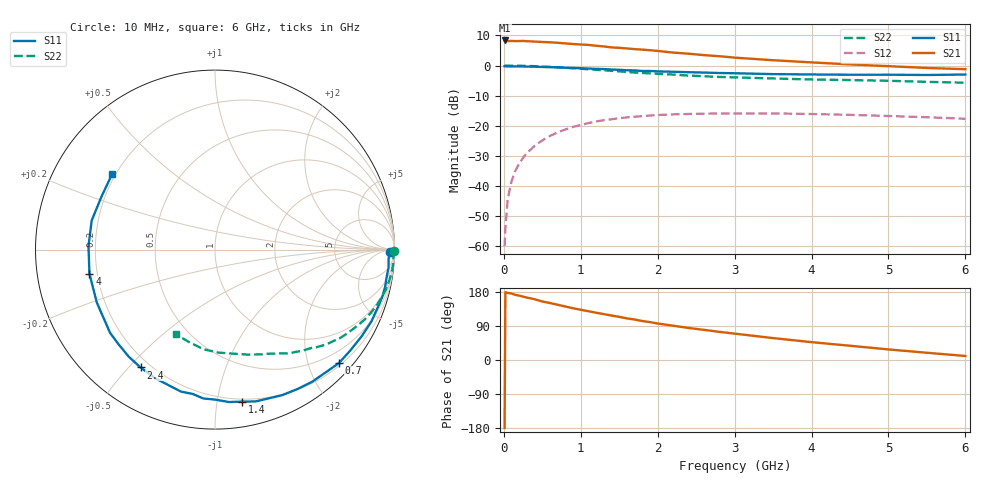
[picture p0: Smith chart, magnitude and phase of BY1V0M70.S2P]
! SIEMENS Small Signal Semiconductors
! BFY420
! Si NPN RF SIEGET Grounded Emitter Transistor in MICRO-X
! VCE = 1 V  IC = 0.7 mA
! Common Emitter S-Parameters:  October  1996
# GHz  S  MA  R  50
!  f  S11  S21  S12  S22
! GHz  MAG  ANG  MAG  ANG  MAG  ANG  MAG  ANG
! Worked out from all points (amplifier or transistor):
!   36 points, 10 MHz to 6 GHz, reference 50 ohm
!   highest |S21| = 8.4 dB at 10 MHz (marker M1)
!   |S21| within 3 dB of that: start of sweep to 1.772 GHz
!   unconditionally stable (mu >= 1): 4.688 GHz to end of sweep
!   at 250 MHz: K = 0.04, MSG = 19.4 dB, |S12| = -30.7 dB
!   at 1.4 GHz: K = 0.22, MSG = 11.9 dB, |S12| = -17.8 dB
!   at 6 GHz: K = 1.34, MAG = 4.7 dB, |S12| = -17.7 dB
!   S11 on the Smith chart (normalised r, x): 10 MHz: 60, -32; 700 MHz: 0.25, -2.55; 1.4 GHz: 0.18, -1.18; 2.4 GHz: 0.16, -0.54; 4 GHz: 0.17, -0.09; 6 GHz: 0.19, +0.32
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0.01  0.9745 -0.8  2.616 -179.4  0.001 107.4  0.9985 -0.3
0.02  0.973 -1.5  2.609 178.7  0.002 85.0  0.9984 -0.6
0.05  0.9682 -3.1  2.555 177.1  0.006 87.8  0.9968 -1.6
0.1  0.9723 -6.1  2.57 175.5  0.012 86.9  0.994 -3.3
0.15  0.9683 -9.1  2.551 171.8  0.0179 83.2  0.9947 -5.0
0.25  0.9691 -15.4  2.57 167.3  0.0293 79.3  0.9896 -8.2
0.4  0.9592 -24.6  2.506 160.4  0.0464 74.1  0.978 -13.1
0.5  0.9487 -30.9  2.469 154.4  0.0572 70.3  0.9652 -16.2
0.7  0.9361 -42.5  2.394 145.7  0.0777 63.1  0.9369 -22.1
0.9  0.9137 -53.8  2.282 136.5  0.0957 55.3  0.9025 -27.6
1.1  0.8933 -65.1  2.206 128.7  0.1109 48.6  0.8685 -32.9
1.4  0.8602 -79.9  2.005 117.3  0.1284 39.4  0.8191 -39.7
1.6  0.8357 -89.9  1.925 109.8  0.1379 33.9  0.7847 -43.9
1.8  0.8137 -98.8  1.842 102.8  0.1447 28.9  0.755 -47.4
2.2  0.7904 -115.1  1.645 90.5  0.1548 19.8  0.7098 -54.6
2.4  0.7766 -122.3  1.576 84.6  0.157 16.1  0.6827 -57.8
2.8  0.7529 -135.6  1.432 74.3  0.1599 9.1  0.6477 -63.7
3.5  0.7215 -155.9  1.228 57.8  0.1607 -0.4  0.6111 -73.1
4  0.7122 -169.1  1.13 47.1  0.1568 -6.0  0.588 -80.3
4.5  0.7053 178.5  1.046 37.6  0.1519 -11.0  0.5747 -87.7
5.5  0.698 154.9  0.914 19.1  0.1387 -17.1  0.5366 -105.0
6  0.7111 143.7  0.871 10.6  0.1306 -18.1  0.52 -114.8
